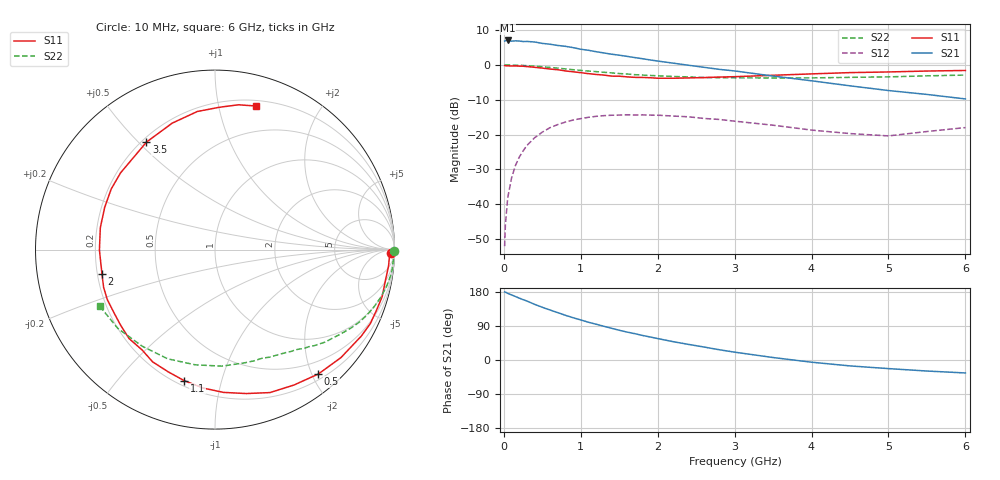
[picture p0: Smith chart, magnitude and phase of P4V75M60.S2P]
! SIEMENS Small Signal Semiconductors
! BFP182
! Si NPN RF Bipolar Junction Transistor in SOT143
! VCE = 0.75 V  IC = 0.6 mA
! Common Emitter S-Parameters:  March  1996
# GHz  S  MA  R  50
!  f  S11  S21  S12  S22
! GHz  MAG  ANG  MAG  ANG  MAG  ANG  MAG  ANG
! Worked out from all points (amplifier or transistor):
!   36 points, 10 MHz to 6 GHz, reference 50 ohm
!   highest |S21| = 7.0 dB at 50 MHz (marker M1)
!   |S21| within 3 dB of that: start of sweep to 1.143 GHz
!   unconditionally stable (mu >= 1): 2.733 GHz to end of sweep
!   at 250 MHz: K = 0.11, MSG = 15.7 dB, |S12| = -24.7 dB
!   at 1.4 GHz: K = 0.54, MSG = 8.8 dB, |S12| = -14.4 dB
!   at 6 GHz: K = 1.46, MAG = 0.1 dB, |S12| = -18.0 dB
!   S11 on the Smith chart (normalised r, x): 10 MHz: 52, -45; 500 MHz: 0.28, -2.10; 1.1 GHz: 0.23, -0.77; 2 GHz: 0.22, -0.10; 3.5 GHz: 0.22, +0.53; 6 GHz: 0.25, +1.30
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0.01  0.9783 -1.1  2.2 179.6  0.0025 87.3  0.9991 -0.4
0.02  0.9728 -1.9  2.233 179.1  0.005 87.3  0.9999 -0.9
0.05  0.9714 -5.3  2.246 175.9  0.0123 87.8  0.9978 -2.1
0.1  0.9651 -10.1  2.194 171.8  0.0237 83.0  0.994 -4.2
0.2  0.9612 -20.6  2.204 163.3  0.0473 76.5  0.9889 -8.4
0.3  0.9469 -30.6  2.175 155.6  0.0697 69.7  0.9763 -12.4
0.4  0.9244 -40.6  2.135 146.9  0.09 63.6  0.9598 -16.3
0.5  0.901 -50.3  2.039 139.1  0.1085 57.2  0.9408 -20.0
0.6  0.8733 -59.8  1.982 132.0  0.1257 51.3  0.921 -23.4
0.8  0.8205 -77.8  1.85 118.0  0.1511 40.5  0.8768 -29.7
1.1  0.7497 -103.3  1.623 99.6  0.1771 26.7  0.817 -37.4
1.5  0.6891 -134.0  1.38 78.5  0.1905 11.6  0.7521 -46.0
1.8  0.6615 -155.1  1.23 64.9  0.1918 3.2  0.7159 -51.4
2  0.6442 -167.7  1.137 56.6  0.1897 -2.1  0.6984 -55.0
2.2  0.6439 -179.7  1.061 48.4  0.1846 -7.0  0.6831 -59.0
3  0.678 140.9  0.82 20.7  0.1558 -20.7  0.6523 -75.2
3.5  0.7103 122.5  0.692 6.5  0.1363 -24.2  0.6505 -86.6
4  0.7438 108.7  0.592 -5.8  0.116 -22.8  0.6513 -99.7
4.5  0.7757 97.3  0.501 -15.6  0.1034 -18.2  0.6632 -113.4
5  0.7929 88.4  0.429 -22.7  0.0957 -6.2  0.6739 -127.0
5.5  0.8174 80.8  0.377 -29.1  0.1107 1.2  0.697 -140.9
6  0.8324 73.9  0.325 -34.2  0.1261 3.9  0.7156 -153.9
